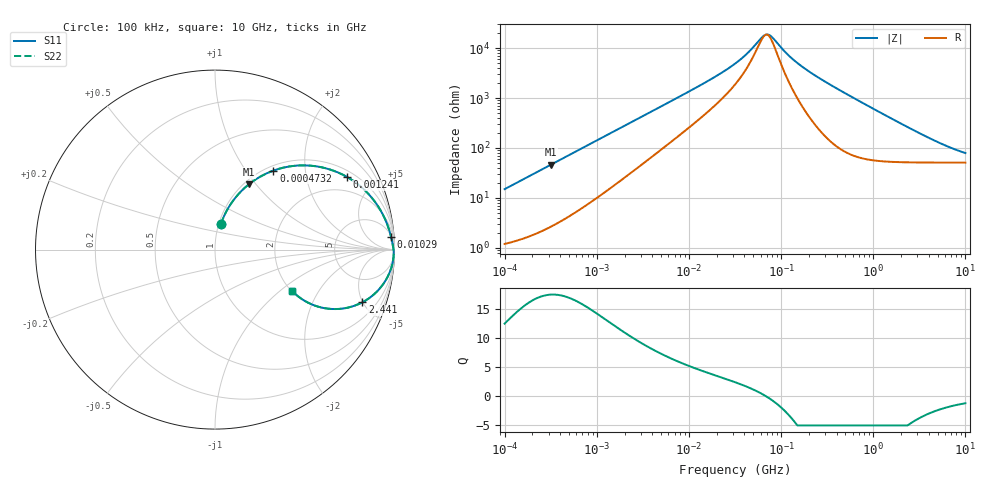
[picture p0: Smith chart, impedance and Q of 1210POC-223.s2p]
# MHz S MA R 50
!Freq  MagS11  AngS11  MagS21  AngS21  MagS12  AngS12  MagS22  AngS22
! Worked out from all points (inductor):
!   801 points, 100 kHz to 10 GHz, reference 50 ohm
!   read as one part in series: L = 23.5 uH near 105.9 kHz
!   highest Q = 17.4 at 316.2 kHz (marker M1), where L = 23.1 uH
!   self-resonance near 67.8 MHz
!   S11 on the Smith chart (normalised r, x): 100 kHz: 1.02, +0.30; 473.2 kHz: 1.08, +1.36; 1.241 MHz: 1.26, +3.48; 10.29 MHz: 6, +27; 2.441 GHz: 2.03, -4.96; 10 GHz: 2.02, -1.21
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0.1  0.1458 77.1  0.9777 -8.4  0.9777 -8.4  0.1458 77.1
0.1883649  0.2626 71.3  0.9489 -15.2  0.9489 -15.2  0.2626 71.3
0.3162278  0.4084 62.7  0.8897 -24.1  0.8897 -24.1  0.4084 62.7
0.4731513  0.5478 53.5  0.8051 -33.1  0.8051 -33.1  0.5478 53.5
0.6878599  0.679 43.7  0.6926 -42.7  0.6926 -42.7  0.679 43.7
1.240938  0.8405 28.7  0.482 -56.9  0.482 -56.9  0.8405 28.7
2.238721  0.9262 17.3  0.2987 -67.2  0.2987 -67.2  0.9262 17.3
4.663908  0.9684 8.7  0.1526 -73.7  0.1526 -73.7  0.9684 8.7
10.29201  0.984 4.0  0.07095 -75.0  0.07095 -75.0  0.984 4.0
20.24184  0.9897 1.9  0.03512 -72.0  0.03512 -72.0  0.9897 1.9
31.62278  0.992 1.1  0.0204 -66.5  0.0204 -66.5  0.992 1.1
43.40103  0.9933 0.6  0.01248 -57.1  0.01248 -57.1  0.9933 0.6
63.09573  0.9944 0.1  0.005886 -18.9  0.005886 -18.9  0.9944 0.1
71.82076  0.9948 -0.1  0.005325 10.5  0.005325 10.5  0.9948 -0.1
80.58422  0.995 -0.2  0.006113 35.5  0.006113 35.5  0.995 -0.2
133.3521  0.9958 -0.9  0.01651 74.9  0.01651 74.9  0.9958 -0.9
217.5204  0.9959 -1.8  0.0323 81.7  0.0323 81.7  0.9959 -1.8
604.2964  0.9885 -5.6  0.09734 80.4  0.09734 80.4  0.9885 -5.6
1474.857  0.9449 -13.1  0.2281 69.6  0.2281 69.6  0.9449 -13.1
2440.619  0.8716 -19.7  0.3442 58.6  0.3442 58.6  0.8716 -19.7
4597.27  0.7047 -27.8  0.4995 41.1  0.4995 41.1  0.7047 -27.8
10000  0.4861 -28.1  0.6156 21.9  0.6156 21.9  0.4861 -28.1
